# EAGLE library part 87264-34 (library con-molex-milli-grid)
RECEPTACAL
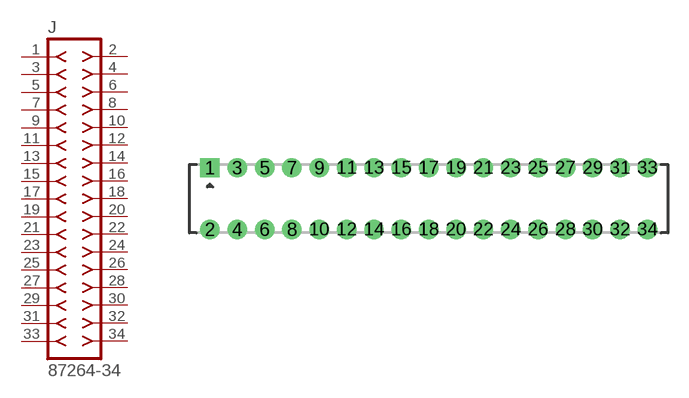
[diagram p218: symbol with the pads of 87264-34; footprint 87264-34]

Designator prefix J

## 87264-34  [87264-34]
1  1  pas
2  2  pas
3  3  pas
4  4  pas
5  5  pas
6  6  pas
7  7  pas
8  8  pas
9  9  pas
10  10  pas
11  11  pas
12  12  pas
13  13  pas
14  14  pas
15  15  pas
16  16  pas
17  17  pas
18  18  pas
19  19  pas
20  20  pas
21  21  pas
22  22  pas
23  23  pas
24  24  pas
25  25  pas
26  26  pas
27  27  pas
28  28  pas
29  29  pas
30  30  pas
31  31  pas
32  32  pas
33  33  pas
34  34  pas

## Footprint 87264-34 (pad centres in mm)
RECEPTACAL Dual Row, Side Entry
drill 0.914 square: 1 -16,2.25
drill 0.914: 2 -16,-2.25; 3 -14,2.25; 4 -14,-2.25; 5 -12,2.25; 6 -12,-2.25; 7 -10,2.25; 8 -10,-2.25; 9 -8,2.25; 10 -8,-2.25; 11 -6,2.25; 12 -6,-2.25; 13 -4,2.25; 14 -4,-2.25; 15 -2,2.25; 16 -2,-2.25; 17 0,2.25; 18 0,-2.25; 19 2,2.25; 20 2,-2.25; 21 4,2.25; 22 4,-2.25; 23 6,2.25; 24 6,-2.25; 25 8,2.25; 26 8,-2.25; 27 10,2.25; 28 10,-2.25; 29 12,2.25; 30 12,-2.25; 31 14,2.25; 32 14,-2.25; 33 16,2.25; 34 16,-2.25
